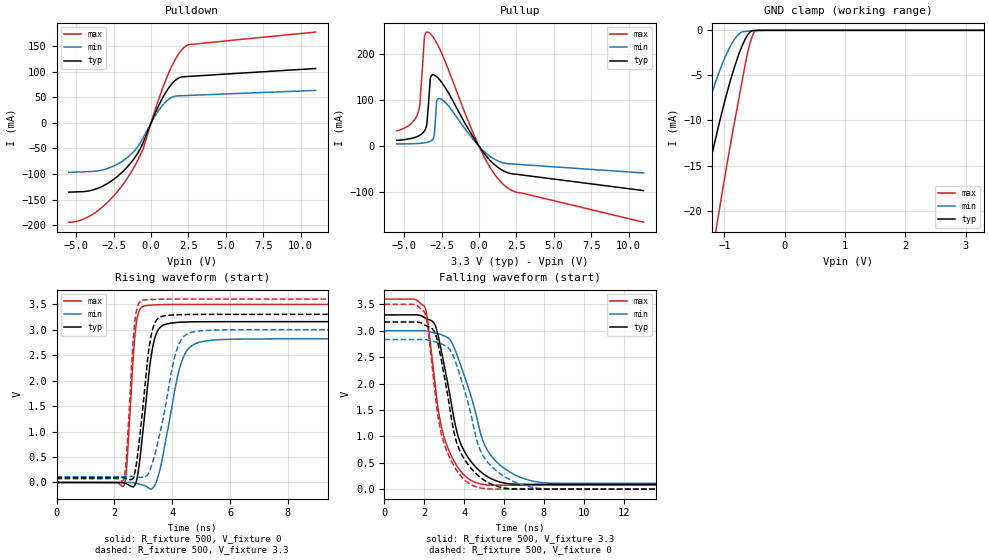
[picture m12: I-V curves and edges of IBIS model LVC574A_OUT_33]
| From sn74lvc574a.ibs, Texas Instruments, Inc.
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[Model]   LVC574A_OUT_33
Model_type  3-state
Enable   Active-Low
Vref =   0
Rref =   500
Cref =   50p
Vmeas =   1.5
| variable   typ   min   max
C_comp   2.56pF   2.43pF   2.80pF
| C_pullup   4.61pF   3.03pF   5.96pF
| C_pulldown   4.13pF   2.21pF   5.88pF
| C_tri-state   2.56pF   2.43pF   2.80pF
[Temperature Range]   40   100   -40
| Ambient temperature   25   85   -40
[Voltage range]   3.3   3   3.6
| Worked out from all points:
|   slope of the pulldown table from 0 to 0.495 V, typ, clamps not added: 15 ohm
|   slope of the pullup table from 0 to 0.495 V, typ, clamps not added: 22.8 ohm
|   GND clamp passes 1 mA (typ) near -0.66 V on its own axis
|   rising waveform, R_fixture 500, V_fixture 0: 20-80 % time 369ps typ, 573ps min, 224ps max; typ from 0 V to 3.16 V
|   falling waveform, R_fixture 500, V_fixture 3.3: 20-80 % time 1.15ns typ, 1.49ns min, 919ps max; typ from 3.3 V to 0.09 V
|   rising waveform, R_fixture 500, V_fixture 3.3: 20-80 % time 362ps typ, 606ps min, 218ps max; typ from 0.09 V to 3.3 V
|   falling waveform, R_fixture 500, V_fixture 0: 20-80 % time 1.1ns typ, 1.37ns min, 899ps max; typ from 3.17 V to 0 V
[GND Clamp]
| LVC574A_OUT_33
|   Voltage   I(typ)   I(min)   I(max)
-5.5V     -186.1mA   -140.6mA   -253.4mA
-1.81V    -33.84mA   -21.6mA    -52.75mA
-1.46V    -21.74mA   -12.6mA    -36.22mA
-1.26V    -15.38mA   -8.042mA   -27.31mA
-1.125V   -11.4mA    -5.326mA   -21.58mA
-925mV    -6.142mA   -2.064mA   -13.62mA
-750mV    -2.451mA   -354.2uA   -7.201mA
-665mV    -1.112mA   -124.4uA   -4.14mA
-595mV    -337.1uA   -87.16uA   -1.918mA
-535mV    -26.65uA   -59.48uA   -605.7uA
-485mV    -6.651uA   -39uA      -60.71uA
3.3V      16.57pA    96.58nA    163.6pA
[Pulldown]
| LVC574A_OUT_33
|   Voltage   I(typ)   I(min)   I(max)
-5.5V     -135.3mA   -96.6mA    -194mA
-4.55V    -134.3mA   -95.71mA   -188.3mA
-3.55V    -127.7mA   -93.82mA   -171.3mA
-2.525V   -110.8mA   -84.64mA   -143.4mA
-1.56V    -85.14mA   -67.05mA   -106.9mA
-985mV    -63.34mA   -50.13mA   -78.32mA
-555mV    -40.07mA   -30.17mA   -52.08mA
280mV     19.39mA    14.25mA    26.09mA
880mV     54.52mA    38.11mA    76.1mA
1.605V    82.57mA    52.16mA    123.2mA
2.27V     90.22mA    53.26mA    148.9mA
11V       106.2mA    63.38mA    177.3mA
[Pullup]
| LVC574A_OUT_33
|   Voltage   I(typ)   I(min)   I(max)
-5.5V     12.83mA    5.219mA    33.28mA
-4.075V   22.04mA    6.078mA    73.25mA
-3.94V    24.41mA    6.393mA    96.75mA
-3.655V   33.2mA     7.444mA    235.4mA
-3.395V   85.64mA    9.296mA    247.5mA
-3.22V    151.4mA    11.73mA    243.2mA
-3V       154.7mA    22.92mA    233.5mA
-2.825V   151mA      98.67mA    223.8mA
-2.615V   143.7mA    103.6mA    210.3mA
115mV     -5.446mA   -3.985mA   -8.053mA
1.695V    -54.3mA    -36.47mA   -84.75mA
11V       -96.08mA   -57.86mA   -164.7mA
[Ramp]
| LVC574A_OUT_33
| variable   typ   min   max
dV/dt_r   1.95/3.86E-10   1.77/5.96E-10   2.14/2.33E-10
dV/dt_f   1.93/1.16E-09   1.73/1.50E-09   2.12/9.22E-10
R_load = 500
[Rising Waveform]
| LVC574A_OUT_33
R_fixture =   500
C_fixture =   0
L_fixture =   0
V_fixture =   0
V_fixture_min = 0
V_fixture_max = 0
|   Time   V(typ)   V(min)   V(max)
0s        224.4pV    4.169nV    1.448nV
2.325ns   -8.06mV    -272.9uV   -64.3mV
2.425ns   -30.13mV   59.11uV    309.9mV
2.74ns    -15.21mV   -13.06mV   3.042V
3.1ns     1.626V     -77.46mV   3.473V
3.315ns   2.628V     -117.7mV   3.484V
3.565ns   3.034V     230.6mV    3.49V
4.355ns   3.147V     2.419V     3.494V
5.31ns    3.156V     2.789V     3.495V
50ns      3.157V     2.821V     3.495V
[Falling Waveform]
| LVC574A_OUT_33
R_fixture =   500
C_fixture =   0
L_fixture =   0
V_fixture =   3.3
V_fixture_min = 3
V_fixture_max = 3.6
|   Time   V(typ)   V(min)   V(max)
0s        3.3V       3V         3.6V
2.005ns   3.25V      2.999V     3.464V
2.505ns   3.135V     2.958V     2.112V
2.835ns   2.658V     2.928V     1.226V
3.285ns   1.78V      2.832V     690.1mV
3.825ns   863.7mV    2.346V     340.2mV
4.885ns   312.9mV    981.9mV    93.83mV
6.08ns    111.3mV    375.7mV    74.71mV
8.2ns     90.28mV    115.3mV    74.1mV
50ns      89.99mV    109.4mV    74.03mV
[Rising Waveform]
| LVC574A_OUT_33
R_fixture =   500
C_fixture =   0
L_fixture =   0
V_fixture =   3.3
V_fixture_min = 3
V_fixture_max = 3.6
|   Time   V(typ)   V(min)   V(max)
0s        89.91mV    109.3mV    74.01mV
2.315ns   93.44mV    114.5mV    41.03mV
2.41ns    78.14mV    117.9mV    469.6mV
2.71ns    204.2mV    113.8mV    3.169V
3.03ns    1.739V     105.7mV    3.584V
3.235ns   2.771V     251.4mV    3.59V
3.46ns    3.191V     688.4mV    3.596V
4.18ns    3.292V     2.644V     3.599V
4.915ns   3.299V     2.973V     3.6V
50ns      3.3V       3V         3.6V
[Falling Waveform]
| LVC574A_OUT_33
R_fixture =   500
C_fixture =   0
L_fixture =   0
V_fixture =   0
V_fixture_min = 0
V_fixture_max = 0
|   Time   V(typ)   V(min)   V(max)
0s        3.166V     2.834V     3.5V
2ns       3.116V     2.834V     3.361V
2.175ns   3.081V     2.824V     3.057V
2.5ns     2.989V     2.793V     1.963V
2.895ns   2.361V     2.745V     988.7mV
3.62ns    888.8mV    2.351V     358.2mV
4.86ns    209mV      695.7mV    19.73mV
6.18ns    12.68mV    203.2mV    558.7uV
8.135ns   341.9uV    4.467mV    87.3uV
50ns      78.01uV    173.8uV    19.88uV
